ORGANIZATION_BLOCK OB 1
BEGIN
	// Test SFC 47: WAIT


	// Zero delay should not wait.
	CALL		SFC 64 ( // Get timestamp
		RET_VAL		:= MD 0
	)
	CALL		SFC 47 (
		WT		:= 0
	)
	__ASSERT==	__STW BIE,	1
	CALL		SFC 64 ( // Get timestamp
		RET_VAL		:= MD 4
	)
	L		MD 4
	L		MD 0
	-D
	UD		DW#16#7FFFFFFF
	__ASSERT<=	__ACCU 1,	10


	// Check short delay.
	CALL		SFC 64 ( // Get timestamp
		RET_VAL		:= MD 0
	)
	CALL		SFC 47 (
		WT		:= 1
	)
	__ASSERT==	__STW BIE,	1
	CALL		SFC 64 ( // Get timestamp
		RET_VAL		:= MD 4
	)
	L		MD 4
	L		MD 0
	-D
	UD		DW#16#7FFFFFFF
	__ASSERT<=	__ACCU 1,	10


	// Check maximum delay.
	CALL		SFC 64 ( // Get timestamp
		RET_VAL		:= MD 0
	)
	CALL		SFC 47 (
		WT		:= 32767
	)
	__ASSERT==	__STW BIE,	1
	CALL		SFC 64 ( // Get timestamp
		RET_VAL		:= MD 4
	)
	L		MD 4
	L		MD 0
	-D
	UD		DW#16#7FFFFFFF
	__ASSERT>=	__ACCU 1,	32
	__ASSERT<=	__ACCU 1,	50


	// Negative delay should not wait.
	CALL		SFC 64 ( // Get timestamp
		RET_VAL		:= MD 0
	)
	CALL		SFC 47 (
		WT		:= -1
	)
	__ASSERT==	__STW BIE,	1
	CALL		SFC 64 ( // Get timestamp
		RET_VAL		:= MD 4
	)
	L		MD 4
	L		MD 0
	-D
	UD		DW#16#7FFFFFFF
	__ASSERT<=	__ACCU 1,	10


	// Negative delay should not wait.
	CALL		SFC 64 ( // Get timestamp
		RET_VAL		:= MD 0
	)
	CALL		SFC 47 (
		WT		:= -32768
	)
	__ASSERT==	__STW BIE,	1
	CALL		SFC 64 ( // Get timestamp
		RET_VAL		:= MD 4
	)
	L		MD 4
	L		MD 0
	-D
	UD		DW#16#7FFFFFFF
	__ASSERT<=	__ACCU 1,	10


	CALL SFC 46 // STOP CPU
END_ORGANIZATION_BLOCK
